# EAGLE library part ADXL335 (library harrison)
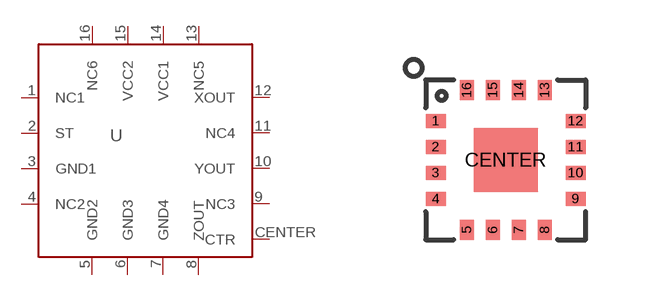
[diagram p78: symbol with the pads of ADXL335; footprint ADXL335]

Designator prefix U

## ADXL335  [ADXL335]
1  NC1  nc
2  ST  in
3  GND1  pwr
4  NC2  nc
5  GND2  pwr
6  GND3  pwr
7  GND4  pwr
8  ZOUT  out
9  NC3  nc
10  YOUT  out
11  NC4  nc
12  XOUT  out
13  NC5  nc
14  VCC1  pwr
15  VCC2  pwr
16  NC6  nc
CENTER  CTR  pas

## Footprint ADXL335 (pad centres in mm)
smd 0.5 x 0.35: 1 -1.75,0.975; 2 -1.75,0.325; 3 -1.75,-0.325; 4 -1.75,-0.975; 9 1.75,-0.975; 10 1.75,-0.325; 11 1.75,0.325; 12 1.75,0.975
smd 0.35 x 0.5: 5 -0.975,-1.75; 6 -0.325,-1.75; 7 0.325,-1.75; 8 0.975,-1.75; 13 0.975,1.75; 14 0.325,1.75; 15 -0.325,1.75; 16 -0.975,1.75
smd 1.6 x 1.6: CENTER 0,0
